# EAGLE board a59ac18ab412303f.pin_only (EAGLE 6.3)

Size 68.58 x 53.34 mm. Coordinates in mm from the lower left corner, seen from the top.
Copper layers (1*16): Top 0.035mm / dielectric 1.5mm / Bottom 0.035mm
Design rules "adafruit": minimum track width 8mil, minimum drill 15.5mil, track to track 8mil, track to pad 8mil, pad to pad 8mil, via to via 8mil, smd to smd 8mil, copper to edge 10mil, drill to drill 8mil, minimum pad ring 10mil, minimum via ring 8mil, stop-mask expansion 2mil, vias tented up to drill 20mil, thermal gap 10mil
Holes 3.2 mm at 15.76,50.75
Holes 2.2 mm at 66.56,35.51

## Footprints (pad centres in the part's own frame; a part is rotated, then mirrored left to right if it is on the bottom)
C025-025X050 = drill 0.813 pad 1.676 octagon: 1 -1.27,0; 2 1.27,0
12-STRIP = drill 1.2 pad 1.676 offset: P$1 0,0; P$11 27.94,0 | drill 1.2 pad 1.676 long: P$2 2.54,0; P$3 5.08,0; P$4 7.62,0; P$5 10.16,0; P$6 12.7,0; P$7 15.24,0; P$8 17.78,0; P$9 20.32,0; P$10 22.86,0; P$12 25.4,0
SO-14NMW = smd 0.635 x 4.445: P$1 -3.048,-3.683; P$2 -1.778,-3.683; P$3 -0.508,-3.683; P$4 0.762,-3.683; P$5 2.032,-3.683; P$6 3.302,-3.683; P$7 4.572,-3.683; P$8 4.572,3.429; P$9 3.302,3.429; P$10 2.032,3.429; P$11 0.762,3.429; P$12 -0.508,3.429; P$13 -1.778,3.429; P$14 -3.048,3.429
1X08-BIG = drill 1.016 pad 1.778 octagon: 1 -8.89,0; 2 -6.35,0; 3 -3.81,0; 4 -1.27,0; 5 1.27,0; 6 3.81,0; 7 6.35,0; 8 8.89,0
1X06-BIG = drill 1.016 pad 1.778 octagon: 1 -6.35,0; 2 -3.81,0; 3 -1.27,0; 4 1.27,0; 5 3.81,0; 6 6.35,0
LED3MM = drill 0.813 pad 1.676 octagon: A -1.27,0; K 1.27,0
ARDUINOR3_ICSP = drill 1 pad 1.676 octagon: 3V 35.56,2.54; 5V 38.1,2.54; A0 50.8,2.54; A1 53.34,2.54; A2 55.88,2.54; A3 58.42,2.54; A4 60.96,2.54; A5 63.5,2.54; AREF 23.876,50.8; D0 63.5,50.8; D1 60.96,50.8; D2 58.42,50.8; D3 55.88,50.8; D4 53.34,50.8; D5 50.8,50.8; D6 48.26,50.8; D7 45.72,50.8; D8 41.656,50.8; D9 39.116,50.8; D10 36.576,50.8; D11 34.036,50.8; D12 31.496,50.8; D13 28.956,50.8; GND 26.416,50.8; GND@1 43.18,2.54; GND@2 40.64,2.54; IOREF 30.48,2.54; RESERVED 27.94,2.54; RESET 33.02,2.54; SCL 18.796,50.8; SDA 21.336,50.8; VIN 45.72,2.54 | drill 1 pad 1.778 octagon: 5V_ICSP 66.167,30.48; GND@3 66.167,25.4; MOSI 66.167,27.94; RESET_ICSP 63.627,25.4; SCK 63.627,27.94 | drill 1 pad 1.778 square: MISO 63.627,30.48
0207/5V = drill 0.813 pad 1.676 octagon: 1 -2.54,0; 2 2.54,0
B3F-10XX = drill 1.016 long: 1 -3.251,2.261; 2 3.251,2.261; 3 -3.251,-2.261; 4 3.251,-2.261
1X10-BIG = drill 1.016 pad 1.778 octagon: 1 -11.43,0; 2 -8.89,0; 3 -6.35,0; 4 -3.81,0; 5 -1.27,0; 6 1.27,0; 7 3.81,0; 8 6.35,0; 9 8.89,0; 10 11.43,0
PERFHOLE = drill 1.1 pad 1.676: 1 0,0
5-STRIP = drill 1 pad 1.676 long: P$1 2.54,0; P$2 5.08,0; P$5 7.62,0 | drill 1 pad 1.676 offset: P$3 0,0; P$4 10.16,0
3-STRIP = drill 1.2 pad 1.676 offset: 1 -2.54,0; P$5 2.54,0 | drill 1.2 pad 1.676 long: P$6 0,0

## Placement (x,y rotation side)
C1  [C025-025X050]  63.67,43.57 0 top
C2  [C025-025X050]  66.66,7.41 90 top
GNDSTRIP1  12-STRIP  [12-STRIP]  56.4,27.89 180 top
GNDSTRIP2  12-STRIP  [12-STRIP]  58.94,10.11 180 top
IC1  SMD-14  [SO-14NMW]  6.36,37.8 0 top
JP1  [1X08-BIG]  36.83,6.35 180 top
JP4  [1X08-BIG]  54.61,46.99 180 top
JP9  [1X06-BIG]  57.15,6.35 0 top
LED1  [LED3MM]  2.62,50.03 270 top
LED2  [LED3MM]  14.87,3.13 270 top
M1  ARDUINO_R3_ICSP  [ARDUINOR3_ICSP]  0,0 0 top
R1  [0207/5V]  9.44,51.32 0 top
R2  [0207/5V]  11.57,4.15 90 top
RESET  Reset  [B3F-10XX]  5.14,3.7 180 top
S1  Reset  [B3F-10XX]  21.6,3.89 0 top
U$1  PINHD-1X10  [1X10-BIG]  30.23,46.99 0 top
U$2  PERFHOLE  [PERFHOLE]  3.06,27.89 0 top
U$3  5-STRIP  [5-STRIP]  66.55,11.43 90 top
U$4  PERFHOLE  [PERFHOLE]  15,6.81 0 top
U$5  3-STRIP  [3-STRIP]  48.78,20.27 90 top
U$6  PERFHOLE  [PERFHOLE]  5.6,27.89 0 top
U$7  PERFHOLE  [PERFHOLE]  10.17,48.98 0 top
U$8  PERFHOLE  [PERFHOLE]  5.6,30.43 0 top
U$9  PERFHOLE  [PERFHOLE]  8.14,27.89 0 top
U$10  3-STRIP  [3-STRIP]  46.24,32.97 90 top
U$11  3-STRIP  [3-STRIP]  46.24,20.27 90 top
U$12  3-STRIP  [3-STRIP]  48.78,32.97 90 top
U$13  3-STRIP  [3-STRIP]  51.19,32.97 90 top
U$14  3-STRIP  [3-STRIP]  51.32,20.27 90 top
U$15  3-STRIP  [3-STRIP]  43.83,32.97 90 top
U$16  PERFHOLE  [PERFHOLE]  26.05,4.02 0 top
U$17  3-STRIP  [3-STRIP]  28.46,32.97 90 top
U$18  3-STRIP  [3-STRIP]  31,20.27 90 top
U$19  PERFHOLE  [PERFHOLE]  8.14,30.43 0 top
U$20  3-STRIP  [3-STRIP]  33.54,32.97 90 top
U$21  3-STRIP  [3-STRIP]  38.62,32.97 90 top
U$22  3-STRIP  [3-STRIP]  36.08,20.27 90 top
U$23  3-STRIP  [3-STRIP]  38.62,20.27 90 top
U$24  5-STRIP  [5-STRIP]  61.47,30.48 90 top
U$25  PERFHOLE  [PERFHOLE]  10.68,27.89 0 top
U$26  3-STRIP  [3-STRIP]  28.46,20.27 90 top
U$27  PERFHOLE  [PERFHOLE]  10.68,30.43 0 top
U$28  3-STRIP  [3-STRIP]  41.16,32.97 90 top
U$29  3-STRIP  [3-STRIP]  31,32.97 90 top
U$30  3-STRIP  [3-STRIP]  36.08,32.97 90 top
U$31  3-STRIP  [3-STRIP]  33.54,20.27 90 top
U$32  3-STRIP  [3-STRIP]  43.7,20.27 90 top
U$33  3-STRIP  [3-STRIP]  41.16,20.27 90 top
U$34  PERFHOLE  [PERFHOLE]  13.22,35.51 90 top
U$35  PERFHOLE  [PERFHOLE]  15.76,35.51 90 top
U$36  [ADAFRUIT_9MM]  10.67,42.67 270 bottom
U$37  PERFHOLE  [PERFHOLE]  13.22,38.05 90 top
U$38  PERFHOLE  [PERFHOLE]  15.76,38.05 90 top
U$39  PERFHOLE  [PERFHOLE]  13.22,40.59 90 top
U$40  PERFHOLE  [PERFHOLE]  15.76,40.59 90 top
U$41  PERFHOLE  [PERFHOLE]  15.76,43.13 90 top
U$43  5-STRIP  [5-STRIP]  61.47,12.7 90 top
VCCSTRIP1  12-STRIP  [12-STRIP]  58.94,43.13 180 top
VCCSTRIP2  12-STRIP  [12-STRIP]  56.4,25.35 180 top

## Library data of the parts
C1 C2 R1 R2 = rcl-ez
GNDSTRIP1 GNDSTRIP2 U$2 U$4-U$35 U$37-U$41 U$43 VCCSTRIP1 VCCSTRIP2 = Atmex
IC1 JP1 JP4 JP9 = carduino
LED1 LED2 M1 U$1 = adafruit
RESET S1 = switch-omron
U$3 = protoshield
U$36 = microbuilder

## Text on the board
tPlace: Digital I/O | Digital I/O | + | ProtoShield v6 | 5V | 14 | SOIC | 5V | 1 | GND | ICSP | 5V | GND | GND | http://www.ladyada.net/make/pshield | Reset | + | Analog In

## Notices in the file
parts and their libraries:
microbuilder: This work is placed in the public domain, and may be freely used for commercial and non-commercial work with the following conditions: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
